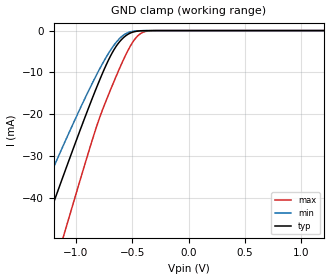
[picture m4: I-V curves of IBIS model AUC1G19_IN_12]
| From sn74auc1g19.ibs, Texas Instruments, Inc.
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[Model]   AUC1G19_IN_12
Model_type  Input
Vinl=0.42
Vinh=0.78
| variable   typ   min   max
C_comp   2.53pF   2.08pF   2.97pF
[Temperature Range]   40   100   -40
| Ambient temperature   25   85   -40
[Voltage range]   1.2   1.1   1.3
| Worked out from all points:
|   GND clamp passes 1 mA (typ) near -0.55 V on its own axis
[GND Clamp]
| AUC1G19_IN_12
|   Voltage   I(typ)   I(min)   I(max)
-3.6V     -226mA     -190mA     -273.7mA
-1.46V    -60.95mA   -48.99mA   -81.11mA
-1.415V   -57.52mA   -46.15mA   -77.01mA
-1.285V   -47.65mA   -38.02mA   -65.13mA
-1.12V    -35.28mA   -27.91mA   -50.04mA
-1.085V   -32.69mA   -25.81mA   -46.84mA
-830mV    -14.47mA   -11.23mA   -24.01mA
-690mV    -5.886mA   -4.537mA   -13.93mA
-570mV    -1.488mA   -934.6uA   -6.46mA
-440mV    -95.43uA   -45.71uA   -982uA
-320mV    -2.85uA    -1.758uA   -25.54uA
1.2V      133.3pA    223.8pA    123.7pA
